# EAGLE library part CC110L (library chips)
The CC110L is a cost optimized sub-1 GHz RF transceiver for the 300–348 MHz, 387–464 MHz, and 779–928 MHz frequency bands.
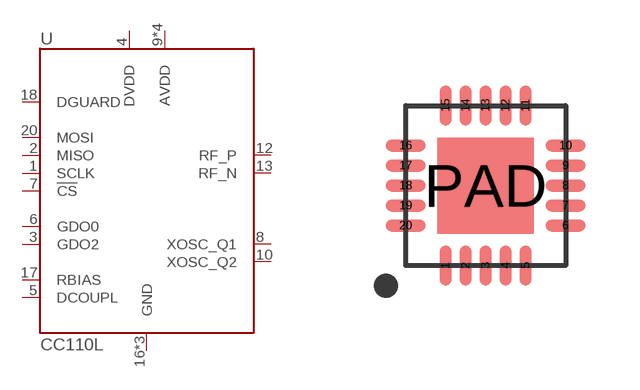
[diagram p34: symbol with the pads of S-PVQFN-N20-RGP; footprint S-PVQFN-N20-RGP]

Designator prefix U

## CC110L (DIGIKEY: 296-35719-1-ND)  [S-PVQFN-N20-RGP]
1  SCLK
2  MISO
3  GDO2
4  DVDD
5  DCOUPL
6  GDO0
7  !CS
8  XOSC_Q1
9  AVDD
10  XOSC_Q2
11  AVDD
12  RF_P
13  RF_N
14  AVDD
15  AVDD
16  GND
17  RBIAS
18  DGUARD
19  GND
20  MOSI
PAD  GND

## Footprint S-PVQFN-N20-RGP (pad centres in mm)
smd 0.3 x 1: 1 -1,-2; 2 -0.5,-2; 3 0,-2; 4 0.5,-2; 5 1,-2; 11 1,2; 12 0.5,2; 13 0,2; 14 -0.5,2; 15 -1,2
smd 1 x 0.3: 6 2,-1; 7 2,-0.5; 8 2,0; 9 2,0.5; 10 2,1; 16 -2,1; 17 -2,0.5; 18 -2,0; 19 -2,-0.5; 20 -2,-1
smd 2.4 x 2.4: PAD 0,0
